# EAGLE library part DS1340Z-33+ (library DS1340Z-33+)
Maxim DS1340Z-33+ Real Time Clock Battery Backup, Calendar, Clock 8-Pin SOIC Source: Datasheet
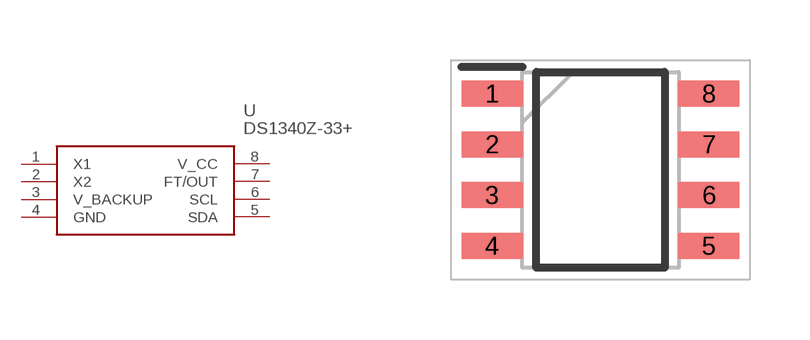
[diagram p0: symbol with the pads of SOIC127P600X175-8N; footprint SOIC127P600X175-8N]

Designator prefix U

## DS1340Z-33+ (Description: Maxim DS1340Z-33+ Real Time Clock Battery Backup, Calendar, Clock 8-Pin SOIC; Height: 1.75mm; Manufacturer_Name: Maxim Integrated; Manufacturer_Part_Number: DS1340Z-33+; Mouser_Part_Number: 700-DS1340Z-33; Mouser_Price-Stock: https://www.mouser.com/Search/Refine.aspx?Keyword=700-DS1340Z-33; RS_Part_Number: 9235839; RS_Price-Stock: https://uk.rs-online.com/web/p/products/9235839)  [SOIC127P600X175-8N]
1  X1  in
2  X2  out
3  V_BACKUP  pwr
4  GND  pwr
5  SDA
6  SCL  in
7  FT/OUT  out
8  V_CC  pwr

## Footprint SOIC127P600X175-8N (pad centres in mm)
8 SO
smd 1.525 x 0.65: 1 -2.712,1.905; 2 -2.712,0.635; 3 -2.712,-0.635; 4 -2.712,-1.905; 5 2.712,-1.905; 6 2.712,-0.635; 7 2.712,0.635; 8 2.712,1.905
